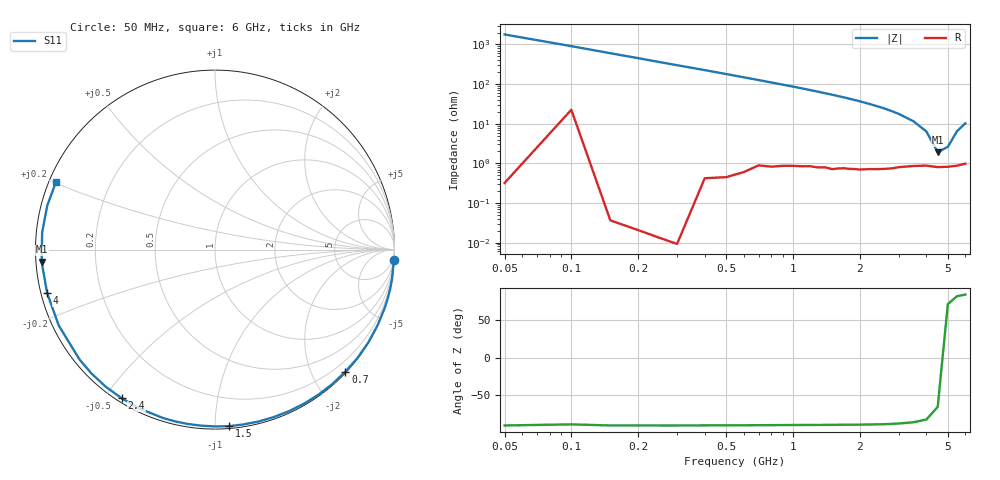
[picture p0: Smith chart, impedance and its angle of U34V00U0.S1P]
! SIEMENS Discrete & RF Semiconductors
! BBY53-02W
! Si Tuning Diode in SCD-80
! VR = 4 V
! S-Parameters:  September  1997
# GHz  S  MA  R  50
!  f  S11
! GHz  MAG  ANG
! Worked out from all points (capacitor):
!   34 points, 50 MHz to 6 GHz, reference 50 ohm
!   read as one part to ground: C = 1.76 pF near 50 MHz
!   lowest |Z| = 1.92 ohm at 4.5 GHz (marker M1)
!   series resonance near 4.706 GHz, so ESL is about 650 pH
!   S11 on the Smith chart (normalised r, x): 50 MHz: 0, -36; 700 MHz: 0.02, -2.53; 1.5 GHz: 0.01, -1.08; 2.4 GHz: 0.01, -0.55; 4 GHz: 0.02, -0.13; 6 GHz: 0.02, +0.20
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0.05  1 -3.2
0.2  1 -12.6
0.3  1 -18.9
0.4  0.9992 -25.0
0.5  0.9987 -31.1
0.6  0.9976 -37.2
0.7  0.9952 -43.1
0.8  0.9944 -48.9
0.9  0.9927 -54.6
1  0.9914 -60.0
1.1  0.9902 -65.4
1.2  0.9887 -70.7
1.3  0.9882 -75.8
1.5  0.9869 -85.5
1.6  0.9852 -90.1
1.8  0.9834 -98.9
2  0.9821 -107.1
2.2  0.9798 -114.9
2.4  0.9783 -122.1
2.6  0.9767 -128.7
2.8  0.9748 -135.0
3  0.9719 -140.9
3.5  0.9679 -154.1
4  0.966 -165.6
4.5  0.9684 -176.0
5  0.9678 174.3
5.5  0.9662 165.3
6  0.9629 156.9
